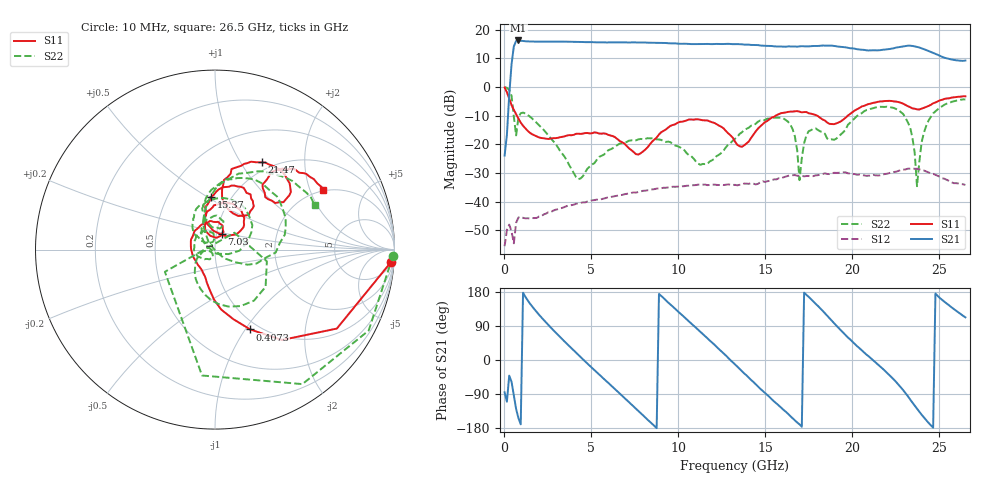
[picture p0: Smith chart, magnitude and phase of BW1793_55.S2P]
!Agilent Technologies,N5242A,MY52422126,A.09.90.01
!Agilent N5242A: A.09.90.01
!Date: Wednesday, September 07, 2016 21:30:09
!Correction: S11(Full 2 Port(1,2))
!S21(Full 2 Port(1,2))
!S12(Full 2 Port(1,2))
!S22(Full 2 Port(1,2))
!S2P File: Measurements: S11, S21, S12, S22:
# Hz S  dB  R 50
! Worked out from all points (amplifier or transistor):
!   201 points, 10 MHz to 26.5 GHz, reference 50 ohm
!   highest |S21| = 16.2 dB at 804.7 MHz (marker M1)
!   |S21| within 3 dB of that: 520.8 MHz to 20.23 GHz (19.71 GHz wide, 190 % of centre)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
!   unconditionally stable (mu >= 1): start of sweep to end of sweep
!   at 4.381 GHz: K = 8.40, MAG = 15.8 dB, |S12| = -40.4 dB
!   at 13.26 GHz: K = 4.47, MAG = 15.1 dB, |S12| = -34.1 dB
!   at 26.5 GHz: K = 3.38, MAG = 13.5 dB, |S12| = -34.1 dB
!   S11 on the Smith chart (normalised r, x): 10 MHz: 7, -26; 407.4 MHz: 0.90, -1.05; 7.03 GHz: 1.06, +0.18; 15.37 GHz: 0.81, +0.52; 21.47 GHz: 0.89, +1.24; 26.5 GHz: 1.95, +2.47
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1e7  -0.16 -4.2  -23.89 -85.3  -55.46 4.3  -0.06 -2.0
4.0735e8  -6.27 -66.3  7.81 -57.1  -50.29 -13.3  -3.03 -95.9
5.398e8  -7.95 -75.3  14.12 -93.3  -54.47 33.1  -10.30 -156.1
8.047e8  -11.02 -90.8  16.22 -153.3  -45.47 18.3  -10.56 -12.7
1.46695e9  -15.97 -110.7  15.86 148.9  -45.83 -10.5  -10.33 -86.1
2.3941e9  -18.00 -143.4  15.84 99.0  -44.11 -25.1  -15.91 -134.5
4.5133e9  -16.23 124.2  15.67 1.7  -40.18 -85.1  -31.08 -118.8
5.8378e9  -16.31 81.9  15.52 -55.0  -38.67 -124.3  -22.87 -133.9
7.02985e9  -20.58 66.7  15.52 -105.9  -37.22 -162.8  -19.15 -173.6
8.88415e9  -16.55 112.3  15.36 174.4  -35.29 133.1  -18.28 124.5
1.100335e10  -11.26 69.3  14.96 85.4  -34.17 54.6  -25.90 98.3
1.3255e10  -19.01 44.1  14.95 -11.5  -34.11 -31.6  -18.04 144.3
1.444705e10  -15.47 108.1  14.62 -63.9  -33.94 -75.0  -12.80 120.3
1.53742e10  -10.63 94.6  14.28 -103.8  -32.47 -109.2  -10.82 86.0
1.66987e10  -8.46 67.9  14.11 -159.4  -30.69 -171.1  -17.26 -2.4
1.77583e10  -9.53 50.5  14.29 154.6  -31.05 145.7  -14.54 91.6
1.921525e10  -12.35 73.4  14.06 84.4  -29.91 84.5  -17.23 100.8
2.14669e10  -5.17 61.8  12.78 -11.9  -30.83 -1.7  -6.96 59.9
2.212915e10  -4.84 49.5  13.22 -39.9  -29.99 -23.8  -6.96 36.0
2.318875e10  -6.68 34.7  14.39 -95.3  -28.47 -74.3  -12.25 -18.6
2.41159e10  -7.26 52.1  13.17 -151.6  -29.11 -129.5  -15.87 115.0
2.65e10  -3.25 29.0  9.21 112.6  -34.15 125.1  -4.34 23.9
